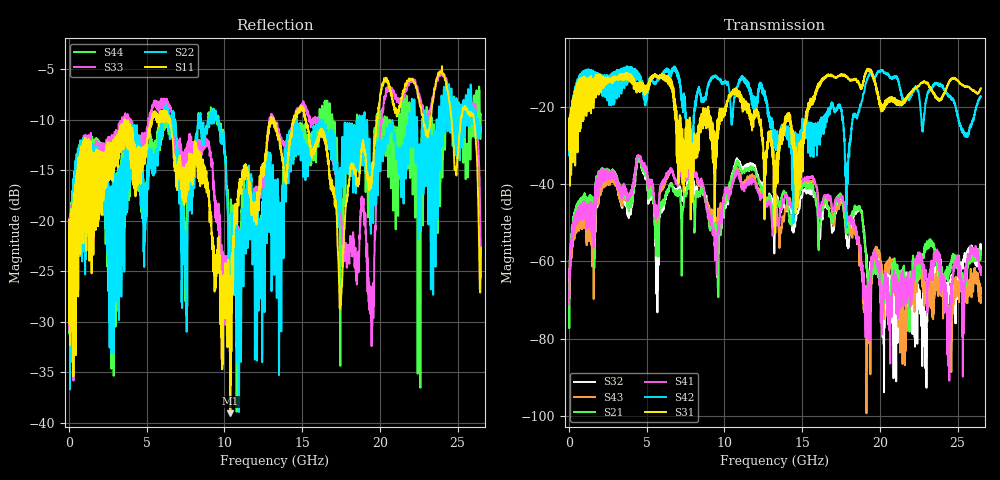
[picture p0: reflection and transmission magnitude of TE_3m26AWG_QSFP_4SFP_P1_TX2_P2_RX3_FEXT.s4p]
!Agilent Technologies,N5222A,MY51421691,A.10.00.00
!Agilent N5222A: A.10.00.00
!Date: Friday, January 30, 2015 12:37:57
!Correction: S11(Full 4 Port(1,2,3,4))
!S12(Full 4 Port(1,2,3,4))
!S13(Full 4 Port(1,2,3,4))
!S14(Full 4 Port(1,2,3,4))
!S21(Full 4 Port(1,2,3,4))
!S22(Full 4 Port(1,2,3,4))
!S23(Full 4 Port(1,2,3,4))
!S24(Full 4 Port(1,2,3,4))
!S31(Full 4 Port(1,2,3,4))
!S32(Full 4 Port(1,2,3,4))
!S33(Full 4 Port(1,2,3,4))
!S34(Full 4 Port(1,2,3,4))
!S41(Full 4 Port(1,2,3,4))
!S42(Full 4 Port(1,2,3,4))
!S43(Full 4 Port(1,2,3,4))
!S44(Full 4 Port(1,2,3,4))
!S4P File: Measurements: <S11,S12,S13,S14>,
!<S21,S22,S23,S24>,
!<S31,S32,S33,S34>,
!<S41,S42,S43,S44>:
# Hz S  dB  R 50.0
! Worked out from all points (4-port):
!   2650 points, 10 MHz to 26.5 GHz, reference 50 ohm
!   strongest paths, dB at 10 MHz, 6.63 GHz, 13.26 GHz, 19.88 GHz, 26.5 GHz:
!     S31: -24.7, -15.5, -42.5, -17.3, -15.3
!     S42: -25.1, -10.6, -28.6, -10.9, -17.3
!     S41: -71.2, -36.8, -47.1, -61.4, -63.6
!     S21: -67.5, -40.0, -47.9, -63.0, -58.1
!     S43: -69.5, -37.0, -43.1, -58.2, -69.4
!     S32: -62.1, -39.9, -48.6, -58.7, -55.8
!   lowest |S11| = -39.1 dB at 10.38 GHz (marker M1), VSWR 1.02, Z = 49.1 + j0.702 ohm
!   |S11| at or under -10 dB: start of sweep to 3.579 GHz; 6.487 GHz to 12.98 GHz (6.491 GHz wide, 66.7 % of centre); 15.24 GHz to 19.79 GHz (4.552 GHz wide, 26 % of centre)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
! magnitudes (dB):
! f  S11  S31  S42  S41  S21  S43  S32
! 10 MHz  -19.9  -24.7  -25.1  -71.2  -67.5  -69.5  -62.1
! 2.19 GHz  -13.5  -12.2  -12.1  -39.2  -38.8  -40.5  -40.3
! 10.38 GHz  -39.1  -17.6  -18.8  -41.7  -39.6  -41.7  -39.5
! 13.3 GHz  -11.1  -36.1  -31.3  -46.6  -45.0  -42.6  -44.8
! 17.87 GHz  -18.0  -12.2  -43.7  -47.7  -51.7  -48.3  -53.7
! 20.93 GHz  -8.7  -18.6  -12.6  -68.1  -60.7  -63.9  -79.2
! 26.5 GHz  -22.6  -15.3  -17.3  -63.6  -58.1  -69.4  -55.8
